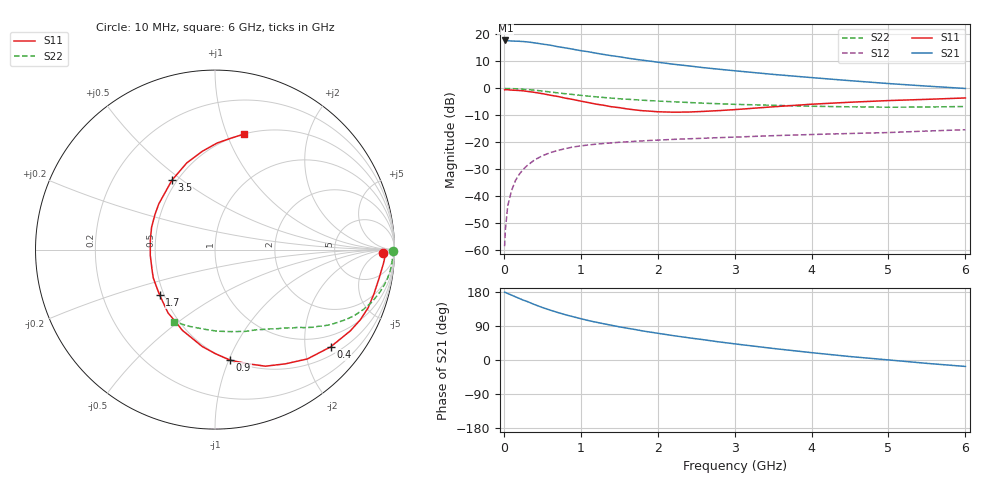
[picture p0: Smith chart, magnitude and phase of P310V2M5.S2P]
! SIEMENS Small Signal Semiconductors
! BFP181
! Si NPN RF Bipolar Junction Transistor in SOT143
! VCE = 10 V  IC = 2.5 mA
! Common Emitter S-Parameters:  March  1996
# GHz  S  MA  R  50
!  f  S11  S21  S12  S22
! GHz  MAG  ANG  MAG  ANG  MAG  ANG  MAG  ANG
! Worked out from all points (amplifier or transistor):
!   36 points, 10 MHz to 6 GHz, reference 50 ohm
!   highest |S21| = 17.7 dB at 20 MHz (marker M1)
!   |S21| within 3 dB of that: start of sweep to 849.7 MHz
!   unconditionally stable (mu >= 1): 2.446 GHz to end of sweep
!   at 250 MHz: K = 0.13, MSG = 23.7 dB, |S12| = -30.1 dB
!   at 1.4 GHz: K = 0.68, MSG = 16.1 dB, |S12| = -20.2 dB
!   at 6 GHz: K = 1.13, MAG = 5.4 dB, |S12| = -15.3 dB
!   S11 on the Smith chart (normalised r, x): 10 MHz: 28, -9; 400 MHz: 0.69, -2.58; 900 MHz: 0.50, -1.01; 1.7 GHz: 0.47, -0.29; 3.5 GHz: 0.47, +0.46; 6 GHz: 0.50, +1.15
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0.01  0.9379 -1.2  7.684 178.7  0.0012 83.0  0.994 -0.4
0.02  0.9484 -2.3  7.691 178.4  0.0024 88.9  0.9911 -0.9
0.05  0.9411 -4.9  7.602 175.4  0.0066 87.4  0.9901 -2.5
0.15  0.9192 -15.7  7.463 166.8  0.0195 79.7  0.9817 -7.3
0.25  0.8992 -25.8  7.341 158.2  0.0314 74.9  0.9623 -12.0
0.3  0.8794 -31.0  7.251 154.7  0.0369 71.1  0.9498 -14.3
0.4  0.8417 -40.1  6.935 146.2  0.0475 66.5  0.9233 -18.3
0.5  0.7975 -49.8  6.594 138.6  0.0564 60.9  0.8913 -22.0
0.6  0.7479 -58.3  6.307 131.8  0.0643 56.5  0.8576 -25.5
0.7  0.7078 -66.6  5.9 125.5  0.0708 52.7  0.8244 -28.3
0.8  0.6589 -74.5  5.604 119.5  0.0767 49.3  0.7948 -30.7
0.9  0.6212 -82.2  5.288 114.2  0.0821 45.9  0.7684 -32.9
1.1  0.5446 -97.5  4.748 104.0  0.0895 41.0  0.7171 -36.6
1.4  0.4558 -119.4  4.02 91.6  0.0979 35.1  0.6587 -41.3
1.7  0.3994 -140.5  3.468 80.6  0.1046 31.4  0.616 -45.1
1.9  0.3783 -155.4  3.188 73.7  0.1086 29.2  0.5921 -47.5
2.2  0.362 -175.2  2.797 64.4  0.1135 26.9  0.5642 -51.3
2.8  0.3874 149.8  2.254 47.7  0.1224 23.1  0.5188 -59.1
3.5  0.4552 121.8  1.812 30.5  0.133 19.5  0.4858 -69.7
4.5  0.5529 97.2  1.386 9.1  0.1459 14.7  0.4548 -88.5
5.5  0.6256 82.1  1.099 -8.9  0.1621 11.5  0.4512 -109.0
6  0.6636 75.9  0.994 -17.0  0.1713 9.1  0.4616 -119.7
